(* Logix 5000 Program export ExtendedLaserCommands; software revision 21.03 *)

TYPE SETTIME :
STRUCT
   cmd : SETTIME_CMD;
   error : DINT;
END_STRUCT
END_TYPE

TYPE SETSYSTEMCOUNTER :
STRUCT
   cmd : SETSYSTEMCOUNTER_CMD;
   error : DINT;
END_STRUCT
END_TYPE

TYPE ExtendedLaserCommands :
STRUCT
   BUFFERCLEAR : NORES_CMD;
   BUFFERDATA : BUFFERDATA;
   BUFFERREVOKE : BUFFERREVOKE;
   GETBUFFERSTATUS : GETBUFFERSTATUS;
   GETCODINGFILE : GETCODINGFILE;
   SETCODINGFILE : SETCODINGFILE;
   GETCODINGLINE : GETINT;
   SETCODINGLINE : SETCODINGLINE;
   GETMSG24 : SIMPLECMD;
   GETMSG25 : MSG25;
   GETSYSTEMCOUNTER : GETSYSTEMCOUNTER;
   SETSYSTEMCOUNTER : SETSYSTEMCOUNTER;
   GETPRINTCOUNTER : GETINT;
   SETMAXCOUNTS : SETMAXCOUNTS;
   GETCO2ONPULSEOFFSET : GETINT;
   GETDATE : GETDATE;
   SETTIME : SETTIME;
   SETDATE : SETDATE;
   priv : LASER_PRIVATE_FIELDS;
END_STRUCT
END_TYPE

TYPE SIMPLECMD :
STRUCT
   cmd : EMPTY_CMD;
   res : LSTRING;
   error : DINT;
END_STRUCT
END_TYPE

TYPE GETDATE :
STRUCT
   cmd : EMPTY_CMD;
   res : GETDATE_RES;
   error : DINT;
END_STRUCT
END_TYPE

TYPE SETCODINGLINE :
STRUCT
   cmd : SETCODINGLINE_CMD;
   error : DINT;
END_STRUCT
END_TYPE

TYPE BUFFERDATA_CMD :
STRUCT
   ID : DINT;
   text1 : LSTRING;
   text2 : LSTRING;
   text3 : LSTRING;
   text4 : LSTRING;
   send : BOOL;
END_STRUCT
END_TYPE

TYPE LSTRING :   // string type
STRUCT
   LEN : DINT;
   DATA : SINT[400];
END_STRUCT
END_TYPE

TYPE SETDATE :
STRUCT
   cmd : SETDATE_CMD;
   error : DINT;
END_STRUCT
END_TYPE

TYPE BUFFERREVOKE :
STRUCT
   cmd : BUFFERREVOKE_CMD;
   error : DINT;
END_STRUCT
END_TYPE

TYPE LASER_PRIVATE_FIELDS :
STRUCT
   data : SINT[808];
   busy : BOOL;
END_STRUCT
END_TYPE

TYPE BUFFERREVOKE_CMD :
STRUCT
   function : LSTRING;
   parameter : DINT;
   send : BOOL;
END_STRUCT
END_TYPE

TYPE MSG25 :
STRUCT
   cmd : EMPTY_CMD;
   res : DINT;
   error : DINT;
END_STRUCT
END_TYPE

TYPE GETBUFFERSTATUS :
STRUCT
   cmd : EMPTY_CMD;
   res : DINT;
   error : DINT;
END_STRUCT
END_TYPE

TYPE GETINT_RES :
STRUCT
   value : DINT;
END_STRUCT
END_TYPE

TYPE SETCODINGFILE_CMD :
STRUCT
   filename : LSTRING;
   nCodes : LSTRING;
   send : BOOL;
END_STRUCT
END_TYPE

TYPE SETTIME_CMD :
STRUCT
   hour : DINT;
   minute : DINT;
   second : DINT;
   send : BOOL;
END_STRUCT
END_TYPE

TYPE EMPTY_CMD :
STRUCT
   send : BOOL;
END_STRUCT
END_TYPE

TYPE GETSYSTEMCOUNTER_CMD :
STRUCT
   id : DINT;
   send : BOOL;
END_STRUCT
END_TYPE

TYPE GETDATE_RES :
STRUCT
   hour : DINT;
   minute : DINT;
   second : DINT;
   year : DINT;
   month : DINT;
   day : DINT;
END_STRUCT
END_TYPE

TYPE GETCODINGFILE :
STRUCT
   cmd : EMPTY_CMD;
   res : GETCODINGFILE_RES;
   error : DINT;
END_STRUCT
END_TYPE

TYPE SETCODINGLINE_CMD :
STRUCT
   value : DINT;
   send : BOOL;
END_STRUCT
END_TYPE

TYPE BUFFERDATA :
STRUCT
   cmd : BUFFERDATA_CMD;
   error : DINT;
END_STRUCT
END_TYPE

TYPE GETSYSTEMCOUNTER_RES :
STRUCT
   id : DINT;
   value : DINT;
END_STRUCT
END_TYPE

TYPE SETSYSTEMCOUNTER_CMD :
STRUCT
   id : DINT;
   value : DINT;
   send : BOOL;
END_STRUCT
END_TYPE

TYPE SETMAXCOUNTS :
STRUCT
   cmd : SETMAXCOUNTS_CMD;
   error : DINT;
END_STRUCT
END_TYPE

TYPE GETINT :
STRUCT
   cmd : EMPTY_CMD;
   res : GETINT_RES;
   error : DINT;
END_STRUCT
END_TYPE

TYPE SETMAXCOUNTS_CMD :
STRUCT
   value : DINT;
   send : BOOL;
END_STRUCT
END_TYPE

TYPE SETDATE_CMD :
STRUCT
   hour : DINT;
   minute : DINT;
   second : DINT;
   year : DINT;
   month : DINT;
   day : DINT;
   send : BOOL;
END_STRUCT
END_TYPE

TYPE GETSYSTEMCOUNTER :
STRUCT
   cmd : GETSYSTEMCOUNTER_CMD;
   res : GETSYSTEMCOUNTER_RES;
   error : DINT;
END_STRUCT
END_TYPE

TYPE GETCODINGFILE_RES :
STRUCT
   filename : LSTRING;
   nCodes : DINT;
END_STRUCT
END_TYPE

TYPE SETCODINGFILE :
STRUCT
   cmd : SETCODINGFILE_CMD;
   error : DINT;
END_STRUCT
END_TYPE

TYPE NORES_CMD :
STRUCT
   cmd : EMPTY_CMD;
   error : DINT;
END_STRUCT
END_TYPE

ADD_ON_INSTRUCTION StrToArr   (* revision 1.0, vendor 1 *)
VAR_IN_OUT
   out : SINT[404]; {required}
   str : LSTRING; {required}
END_VAR
VAR_OUTPUT
   size : DINT; {access Read Only, required}
END_VAR

ROUTINE Logic   (* ladder *)
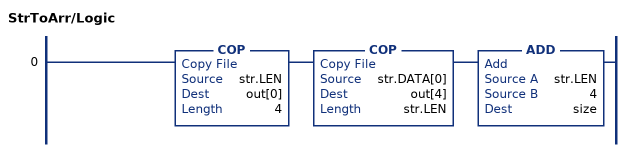
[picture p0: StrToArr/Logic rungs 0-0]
   0: COP(str.LEN,out[0],4)COP(str.DATA[0],out[4],str.LEN)ADD(str.LEN,4,size);
END_ROUTINE
END_ADD_ON_INSTRUCTION

ADD_ON_INSTRUCTION AppendStrs   (* revision 1.0, vendor 1 *)
VAR_IN_OUT
   str1 : LSTRING; {required}
   str2 : LSTRING; {required}
   out : SINT[808]; {required}
END_VAR
VAR_OUTPUT
   size : DINT; {access Read Only, required}
END_VAR
VAR
   cpy : StrToArr; {access None}
   n : DINT; {access None}
   offset : DINT; {access None}
   buf : SINT[404]; {access None}
END_VAR

ROUTINE Logic   (* ladder *)
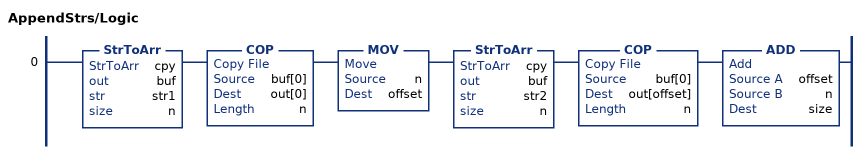
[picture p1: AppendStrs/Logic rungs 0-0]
   0: StrToArr(cpy,buf,str1,n)COP(buf[0],out[0],n)MOV(n,offset)StrToArr(cpy,buf,str2,n)COP(buf[0],out[offset],n)ADD(offset,n,size);
END_ROUTINE
END_ADD_ON_INSTRUCTION

ADD_ON_INSTRUCTION AppendStrs5   (* revision 1.0, vendor 1 *)
VAR_IN_OUT
   str1 : LSTRING; {required}
   str2 : LSTRING; {required}
   str3 : LSTRING; {required}
   str4 : LSTRING; {required}
   str5 : LSTRING; {required}
   out : SINT[808]; {required}
END_VAR
VAR_OUTPUT
   size : DINT; {access Read Only, required}
END_VAR
VAR_INPUT
   number_of_strings : DINT; {required}
   offset : DINT; {required}
END_VAR
VAR
   cpy : StrToArr; {access None}
   n : DINT; {access None}
   buf : SINT[404]; {access None}
END_VAR

ROUTINE Logic   (* ladder *)
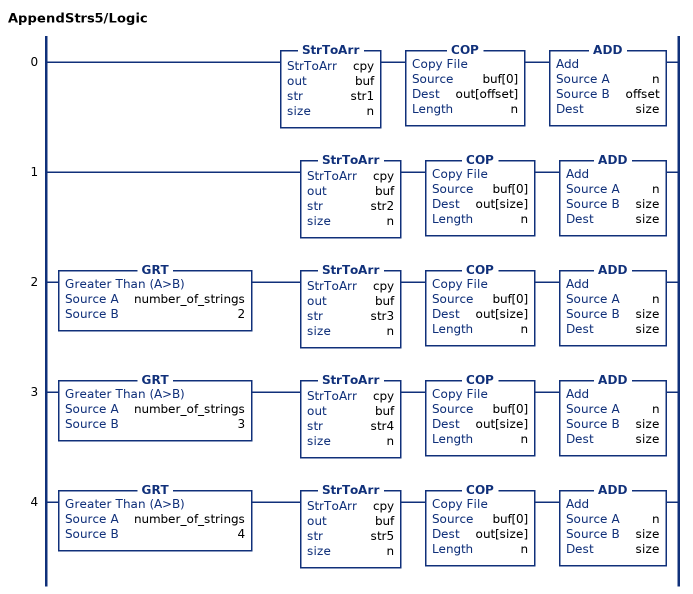
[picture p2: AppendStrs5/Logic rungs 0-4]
   0: StrToArr(cpy,buf,str1,n)COP(buf[0],out[offset],n)ADD(n,offset,size);
   1: StrToArr(cpy,buf,str2,n)COP(buf[0],out[size],n)ADD(n,size,size);
   2: GRT(number_of_strings,2)StrToArr(cpy,buf,str3,n)COP(buf[0],out[size],n)ADD(n,size,size);
   3: GRT(number_of_strings,3)StrToArr(cpy,buf,str4,n)COP(buf[0],out[size],n)ADD(n,size,size);
   4: GRT(number_of_strings,4)StrToArr(cpy,buf,str5,n)COP(buf[0],out[size],n)ADD(n,size,size);
END_ROUTINE
END_ADD_ON_INSTRUCTION

ADD_ON_INSTRUCTION ArrToStr   (* revision 1.0, vendor 1 *)
VAR_IN_OUT
   arr : SINT[404]; {required}
   out : LSTRING; {required}
END_VAR

ROUTINE Logic   (* ladder *)
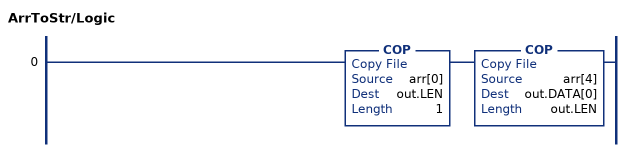
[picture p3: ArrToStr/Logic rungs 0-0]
   0: COP(arr[0],out.LEN,1)COP(arr[4],out.DATA[0],out.LEN);
END_ROUTINE
END_ADD_ON_INSTRUCTION

VAR_GLOBAL   (* controller tags *)
   Domino_internal_getprintcounter : MESSAGE;
        MessageParameters(MessageType := CIP Generic, ConnectedFlag := 2, ConnectionPath := DFSeries, ServiceCode := 16#0057, ObjectType := 16#0065, TargetObject := 1, LocalElement := DFSeriesExtended.priv, DestinationTag := DFSeriesExtended.priv)
   Domino_internal_setcodingline : MESSAGE;
        MessageParameters(MessageType := CIP Generic, RequestedLength := 4, ConnectedFlag := 2, ConnectionPath := DFSeries, ServiceCode := 16#0052, ObjectType := 16#0065, TargetObject := 1, LocalElement := DFSeriesExtended.priv, DestinationTag := DFSeriesExtended.priv)
   Domino_internal_setdate : MESSAGE;
        MessageParameters(MessageType := CIP Generic, RequestedLength := 24, ConnectedFlag := 2, ConnectionPath := DFSeries, ServiceCode := 16#005c, ObjectType := 16#0065, TargetObject := 1, LocalElement := DFSeriesExtended.priv, DestinationTag := DFSeriesExtended.priv)
   Domino_internal_getMSG25 : MESSAGE;
        MessageParameters(MessageType := CIP Generic, ConnectedFlag := 2, ConnectionPath := DFSeries, ServiceCode := 16#0054, ObjectType := 16#0065, TargetObject := 1, LocalElement := DFSeriesExtended.priv, DestinationTag := DFSeriesExtended.priv)
   Domino_internal_setcodingfile : MESSAGE;
        MessageParameters(MessageType := CIP Generic, RequestedLength := 1, ConnectedFlag := 2, ConnectionPath := DFSeries, ServiceCode := 16#0050, ObjectType := 16#0065, TargetObject := 1, LocalElement := DFSeriesExtended.priv, DestinationTag := DFSeriesExtended.priv)
   Domino_internal_setmaxcounts : MESSAGE;
        MessageParameters(MessageType := CIP Generic, RequestedLength := 4, ConnectedFlag := 2, ConnectionPath := DFSeries, ServiceCode := 16#0058, ObjectType := 16#0065, TargetObject := 1, LocalElement := DFSeriesExtended.priv, DestinationTag := DFSeriesExtended.priv)
   Domino_internal_getcodingfile : MESSAGE;
        MessageParameters(MessageType := CIP Generic, ConnectedFlag := 2, ConnectionPath := DFSeries, ServiceCode := 16#004f, ObjectType := 16#0065, TargetObject := 1, LocalElement := DFSeriesExtended.priv, DestinationTag := DFSeriesExtended.priv)
   Domino_internal_setsystemcounter : MESSAGE;
        MessageParameters(MessageType := CIP Generic, RequestedLength := 8, ConnectedFlag := 2, ConnectionPath := DFSeries, ServiceCode := 16#0056, ObjectType := 16#0065, TargetObject := 1, LocalElement := DFSeriesExtended.priv, DestinationTag := DFSeriesExtended.priv)
   Domino_internal_bufferclear : MESSAGE;
        MessageParameters(MessageType := CIP Generic, ConnectedFlag := 2, ConnectionPath := DFSeries, ServiceCode := 16#004b, ObjectType := 16#0065, TargetObject := 1, LocalElement := DFSeriesExtended.priv, DestinationTag := DFSeriesExtended.priv)
   DFSeriesExtended : ExtendedLaserCommands;
   Domino_internal_getcodingline : MESSAGE;
        MessageParameters(MessageType := CIP Generic, ConnectedFlag := 2, ConnectionPath := DFSeries, ServiceCode := 16#0051, ObjectType := 16#0065, TargetObject := 1, LocalElement := DFSeriesExtended.priv, DestinationTag := DFSeriesExtended.priv)
   Domino_internal_getco2onpulseoffset : MESSAGE;
        MessageParameters(MessageType := CIP Generic, ConnectedFlag := 2, ConnectionPath := DFSeries, ServiceCode := 16#0059, ObjectType := 16#0065, TargetObject := 1, LocalElement := DFSeriesExtended.priv, DestinationTag := DFSeriesExtended.priv)
   Domino_internal_getbufferstatus : MESSAGE;
        MessageParameters(MessageType := CIP Generic, ConnectedFlag := 2, ConnectionPath := DFSeries, ServiceCode := 16#004e, ObjectType := 16#0065, TargetObject := 1, LocalElement := DFSeriesExtended.priv, DestinationTag := DFSeriesExtended.priv)
   Domino_internal_bufferdata : MESSAGE;
        MessageParameters(MessageType := CIP Generic, RequestedLength := 1, ConnectedFlag := 2, ConnectionPath := DFSeries, ServiceCode := 16#004c, ObjectType := 16#0065, TargetObject := 1, LocalElement := DFSeriesExtended.priv, DestinationTag := DFSeriesExtended.priv)
   Domino_internal_getdate : MESSAGE;
        MessageParameters(MessageType := CIP Generic, ConnectedFlag := 2, ConnectionPath := DFSeries, ServiceCode := 16#005a, ObjectType := 16#0065, TargetObject := 1, LocalElement := DFSeriesExtended.priv, DestinationTag := DFSeriesExtended.priv)
   Domino_internal_settime : MESSAGE;
        MessageParameters(MessageType := CIP Generic, RequestedLength := 12, ConnectedFlag := 2, ConnectionPath := DFSeries, ServiceCode := 16#005b, ObjectType := 16#0065, TargetObject := 1, LocalElement := DFSeriesExtended.priv, DestinationTag := DFSeriesExtended.priv)
   Domino_internal_bufferrevoke : MESSAGE;
        MessageParameters(MessageType := CIP Generic, RequestedLength := 1, ConnectedFlag := 2, ConnectionPath := DFSeries, ServiceCode := 16#004d, ObjectType := 16#0065, TargetObject := 1, LocalElement := DFSeriesExtended.priv, DestinationTag := DFSeriesExtended.priv)
   Domino_internal_getsystemcounter : MESSAGE;
        MessageParameters(MessageType := CIP Generic, RequestedLength := 4, ConnectedFlag := 2, ConnectionPath := DFSeries, ServiceCode := 16#0055, ObjectType := 16#0065, TargetObject := 1, LocalElement := DFSeriesExtended.priv, DestinationTag := DFSeriesExtended.priv)
   Domino_internal_getMSG24 : MESSAGE;
        MessageParameters(MessageType := CIP Generic, ConnectedFlag := 2, ConnectionPath := DFSeries, ServiceCode := 16#0053, ObjectType := 16#0065, TargetObject := 1, LocalElement := DFSeriesExtended.priv, DestinationTag := DFSeriesExtended.priv)
END_VAR

PROGRAM ExtendedLaserCommands   (* main routine Main *)
VAR
   app : AppendStrs;
   app5 : AppendStrs5;
   toArr : StrToArr;
   toStr : ArrToStr;
END_VAR

ROUTINE Main   (* ladder *)
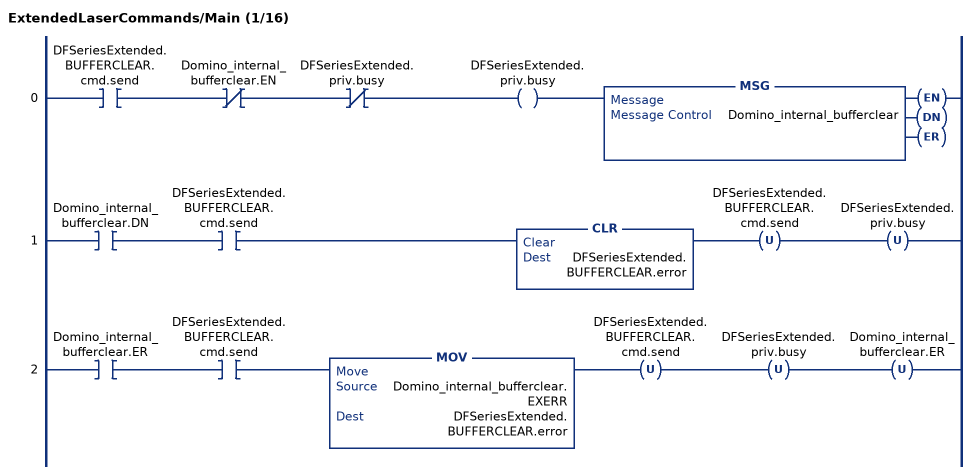
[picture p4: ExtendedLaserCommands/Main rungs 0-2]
   0: XIC(DFSeriesExtended.BUFFERCLEAR.cmd.send)XIO(Domino_internal_bufferclear.EN)XIO(DFSeriesExtended.priv.busy)OTE(DFSeriesExtended.priv.busy)MSG(Domino_internal_bufferclear);
   1: XIC(Domino_internal_bufferclear.DN)XIC(DFSeriesExtended.BUFFERCLEAR.cmd.send)CLR(DFSeriesExtended.BUFFERCLEAR.error)OTU(DFSeriesExtended.BUFFERCLEAR.cmd.send)OTU(DFSeriesExtended.priv.busy);
   2: XIC(Domino_internal_bufferclear.ER)XIC(DFSeriesExtended.BUFFERCLEAR.cmd.send)MOV(Domino_internal_bufferclear.EXERR,DFSeriesExtended.BUFFERCLEAR.error)OTU(DFSeriesExtended.BUFFERCLEAR.cmd.send)OTU(DFSeriesExtended.priv.busy)OTU(Domino_internal_bufferclear.ER);
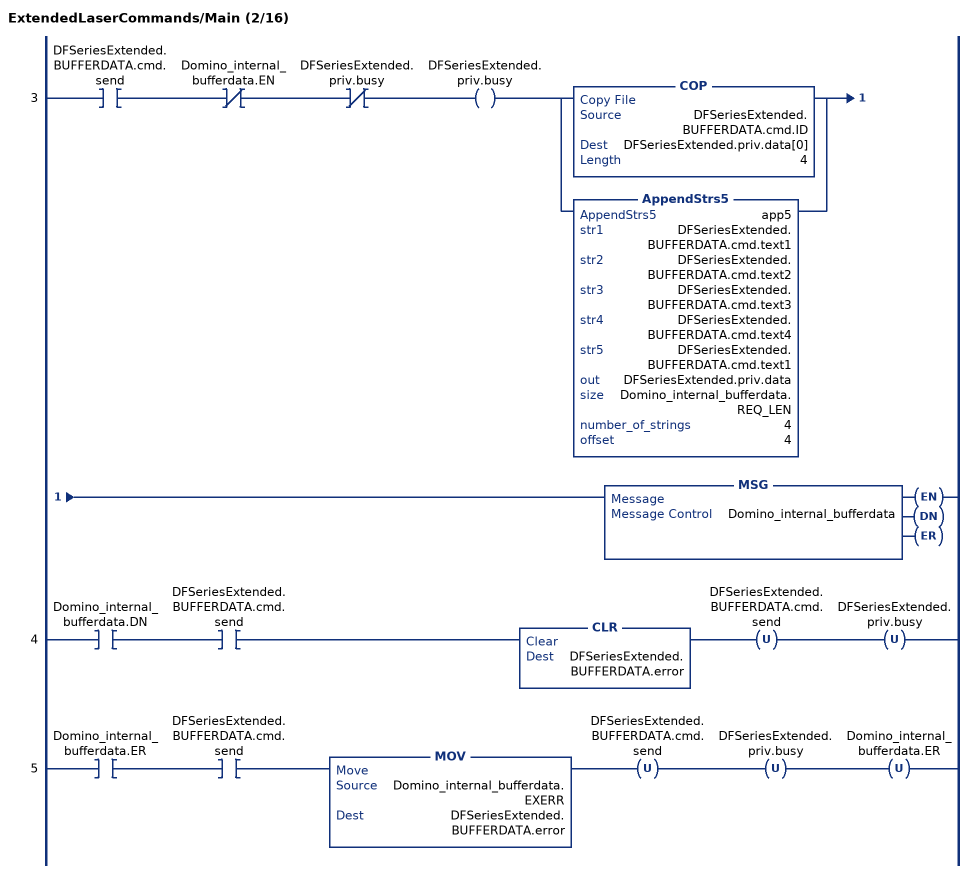
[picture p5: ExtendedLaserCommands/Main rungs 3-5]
   3: XIC(DFSeriesExtended.BUFFERDATA.cmd.send)XIO(Domino_internal_bufferdata.EN)XIO(DFSeriesExtended.priv.busy)OTE(DFSeriesExtended.priv.busy)[COP(DFSeriesExtended.BUFFERDATA.cmd.ID,DFSeriesExtended.priv.data[0],4) ,AppendStrs5(app5,DFSeriesExtended.BUFFERDATA.cmd.text1,DFSeriesExtended.BUFFERDATA.cmd.text2,DFSeriesExtended.BUFFERDATA.cmd.text3,DFSeriesExtended.BUFFERDATA.cmd.text4,DFSeriesExtended.BUFFERDATA.cmd.text1,DFSeriesExtended.priv.data,Domino_internal_bufferdata.REQ_LEN,4,4) ]MSG(Domino_internal_bufferdata);
   4: XIC(Domino_internal_bufferdata.DN)XIC(DFSeriesExtended.BUFFERDATA.cmd.send)CLR(DFSeriesExtended.BUFFERDATA.error)OTU(DFSeriesExtended.BUFFERDATA.cmd.send)OTU(DFSeriesExtended.priv.busy);
   5: XIC(Domino_internal_bufferdata.ER)XIC(DFSeriesExtended.BUFFERDATA.cmd.send)MOV(Domino_internal_bufferdata.EXERR,DFSeriesExtended.BUFFERDATA.error)OTU(DFSeriesExtended.BUFFERDATA.cmd.send)OTU(DFSeriesExtended.priv.busy)OTU(Domino_internal_bufferdata.ER);
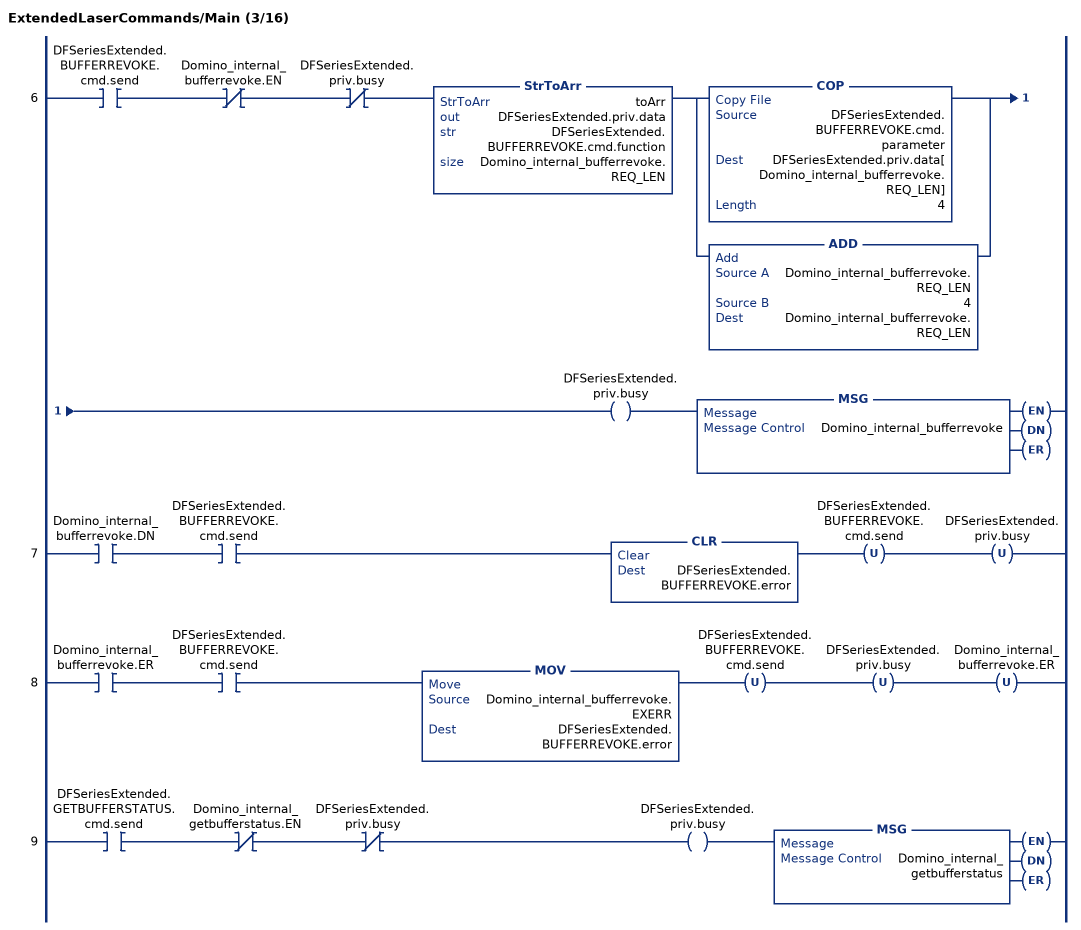
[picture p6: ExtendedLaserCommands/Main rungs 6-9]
   6: XIC(DFSeriesExtended.BUFFERREVOKE.cmd.send)XIO(Domino_internal_bufferrevoke.EN)XIO(DFSeriesExtended.priv.busy)StrToArr(toArr,DFSeriesExtended.priv.data,DFSeriesExtended.BUFFERREVOKE.cmd.function,Domino_internal_bufferrevoke.REQ_LEN)[COP(DFSeriesExtended.BUFFERREVOKE.cmd.parameter,DFSeriesExtended.priv.data[Domino_internal_bufferrevoke.REQ_LEN],4) ,ADD(Domino_internal_bufferrevoke.REQ_LEN,4,Domino_internal_bufferrevoke.REQ_LEN) ]OTE(DFSeriesExtended.priv.busy)MSG(Domino_internal_bufferrevoke);
   7: XIC(Domino_internal_bufferrevoke.DN)XIC(DFSeriesExtended.BUFFERREVOKE.cmd.send)CLR(DFSeriesExtended.BUFFERREVOKE.error)OTU(DFSeriesExtended.BUFFERREVOKE.cmd.send)OTU(DFSeriesExtended.priv.busy);
   8: XIC(Domino_internal_bufferrevoke.ER)XIC(DFSeriesExtended.BUFFERREVOKE.cmd.send)MOV(Domino_internal_bufferrevoke.EXERR,DFSeriesExtended.BUFFERREVOKE.error)OTU(DFSeriesExtended.BUFFERREVOKE.cmd.send)OTU(DFSeriesExtended.priv.busy)OTU(Domino_internal_bufferrevoke.ER);
   9: XIC(DFSeriesExtended.GETBUFFERSTATUS.cmd.send)XIO(Domino_internal_getbufferstatus.EN)XIO(DFSeriesExtended.priv.busy)OTE(DFSeriesExtended.priv.busy)MSG(Domino_internal_getbufferstatus);
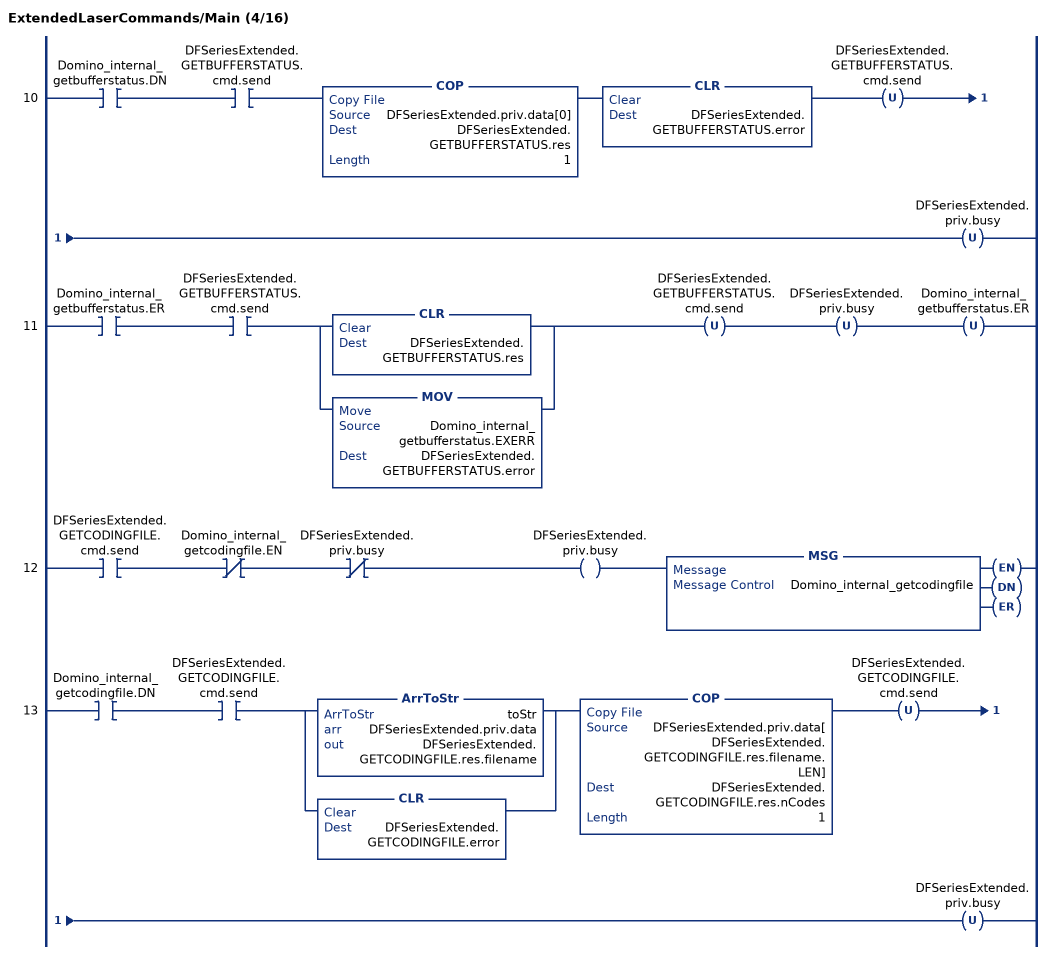
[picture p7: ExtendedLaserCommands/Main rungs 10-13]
   10: XIC(Domino_internal_getbufferstatus.DN)XIC(DFSeriesExtended.GETBUFFERSTATUS.cmd.send)COP(DFSeriesExtended.priv.data[0],DFSeriesExtended.GETBUFFERSTATUS.res,1)CLR(DFSeriesExtended.GETBUFFERSTATUS.error)OTU(DFSeriesExtended.GETBUFFERSTATUS.cmd.send)OTU(DFSeriesExtended.priv.busy);
   11: XIC(Domino_internal_getbufferstatus.ER)XIC(DFSeriesExtended.GETBUFFERSTATUS.cmd.send)[CLR(DFSeriesExtended.GETBUFFERSTATUS.res) ,MOV(Domino_internal_getbufferstatus.EXERR,DFSeriesExtended.GETBUFFERSTATUS.error) ]OTU(DFSeriesExtended.GETBUFFERSTATUS.cmd.send)OTU(DFSeriesExtended.priv.busy)OTU(Domino_internal_getbufferstatus.ER);
   12: XIC(DFSeriesExtended.GETCODINGFILE.cmd.send)XIO(Domino_internal_getcodingfile.EN)XIO(DFSeriesExtended.priv.busy)OTE(DFSeriesExtended.priv.busy)MSG(Domino_internal_getcodingfile);
   13: XIC(Domino_internal_getcodingfile.DN)XIC(DFSeriesExtended.GETCODINGFILE.cmd.send)[ArrToStr(toStr,DFSeriesExtended.priv.data,DFSeriesExtended.GETCODINGFILE.res.filename) ,CLR(DFSeriesExtended.GETCODINGFILE.error) ]COP(DFSeriesExtended.priv.data[DFSeriesExtended.GETCODINGFILE.res.filename.LEN],DFSeriesExtended.GETCODINGFILE.res.nCodes,1)OTU(DFSeriesExtended.GETCODINGFILE.cmd.send)OTU(DFSeriesExtended.priv.busy);
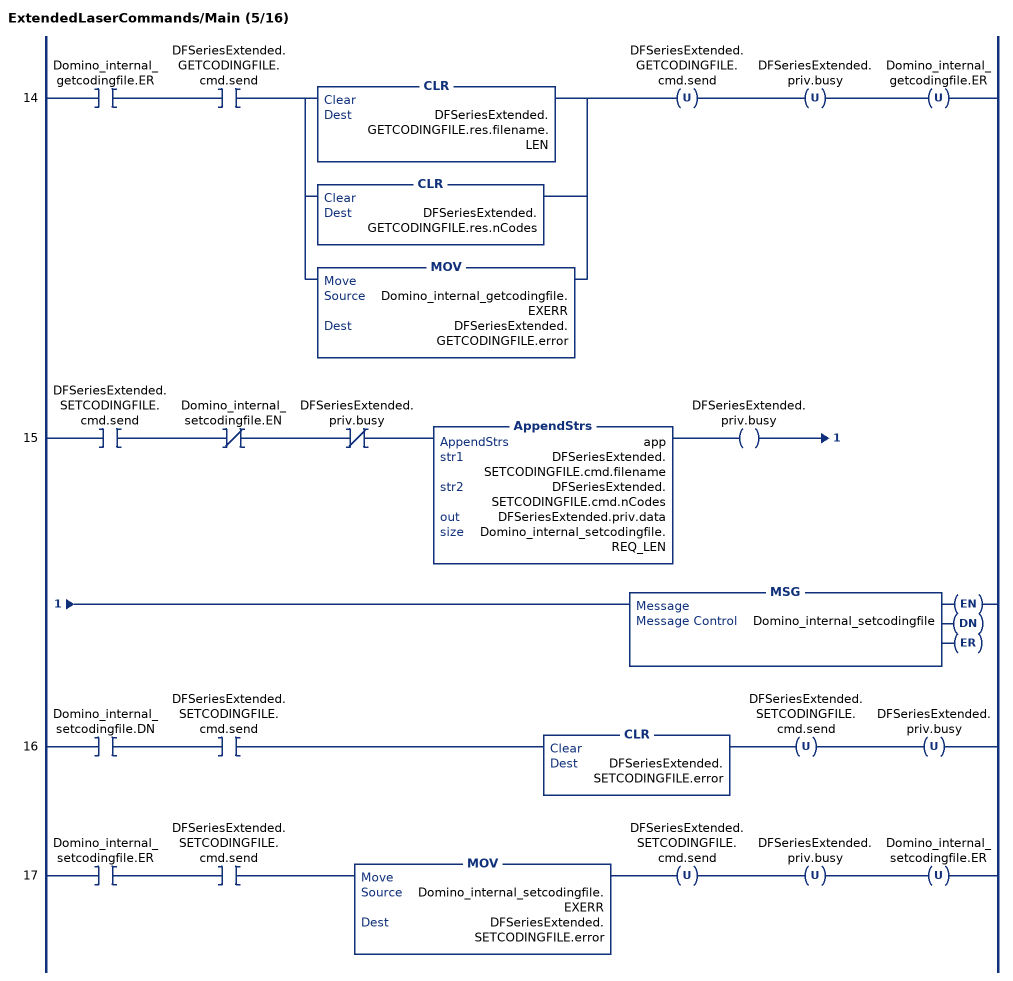
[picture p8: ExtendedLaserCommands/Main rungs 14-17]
   14: XIC(Domino_internal_getcodingfile.ER)XIC(DFSeriesExtended.GETCODINGFILE.cmd.send)[CLR(DFSeriesExtended.GETCODINGFILE.res.filename.LEN) ,CLR(DFSeriesExtended.GETCODINGFILE.res.nCodes) ,MOV(Domino_internal_getcodingfile.EXERR,DFSeriesExtended.GETCODINGFILE.error) ]OTU(DFSeriesExtended.GETCODINGFILE.cmd.send)OTU(DFSeriesExtended.priv.busy)OTU(Domino_internal_getcodingfile.ER);
   15: XIC(DFSeriesExtended.SETCODINGFILE.cmd.send)XIO(Domino_internal_setcodingfile.EN)XIO(DFSeriesExtended.priv.busy)AppendStrs(app,DFSeriesExtended.SETCODINGFILE.cmd.filename,DFSeriesExtended.SETCODINGFILE.cmd.nCodes,DFSeriesExtended.priv.data,Domino_internal_setcodingfile.REQ_LEN)OTE(DFSeriesExtended.priv.busy)MSG(Domino_internal_setcodingfile);
   16: XIC(Domino_internal_setcodingfile.DN)XIC(DFSeriesExtended.SETCODINGFILE.cmd.send)CLR(DFSeriesExtended.SETCODINGFILE.error)OTU(DFSeriesExtended.SETCODINGFILE.cmd.send)OTU(DFSeriesExtended.priv.busy);
   17: XIC(Domino_internal_setcodingfile.ER)XIC(DFSeriesExtended.SETCODINGFILE.cmd.send)MOV(Domino_internal_setcodingfile.EXERR,DFSeriesExtended.SETCODINGFILE.error)OTU(DFSeriesExtended.SETCODINGFILE.cmd.send)OTU(DFSeriesExtended.priv.busy)OTU(Domino_internal_setcodingfile.ER);
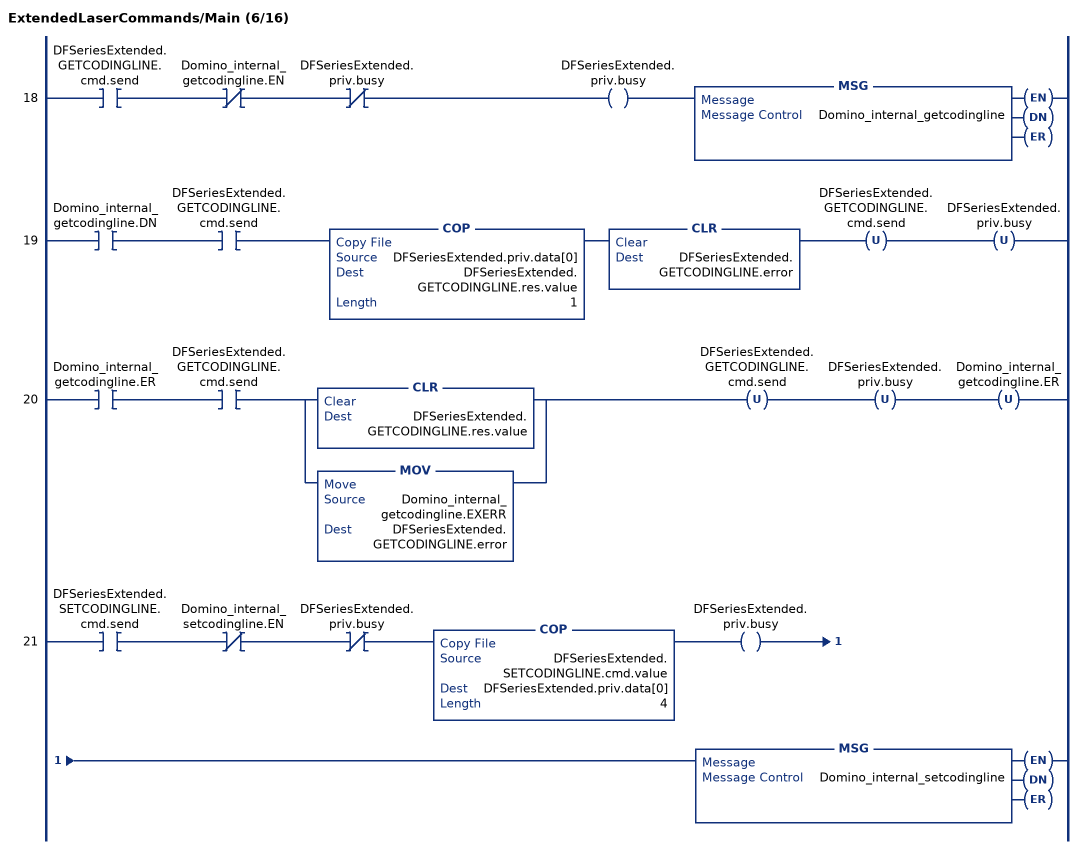
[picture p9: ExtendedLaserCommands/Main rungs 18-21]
   18: XIC(DFSeriesExtended.GETCODINGLINE.cmd.send)XIO(Domino_internal_getcodingline.EN)XIO(DFSeriesExtended.priv.busy)OTE(DFSeriesExtended.priv.busy)MSG(Domino_internal_getcodingline);
   19: XIC(Domino_internal_getcodingline.DN)XIC(DFSeriesExtended.GETCODINGLINE.cmd.send)COP(DFSeriesExtended.priv.data[0],DFSeriesExtended.GETCODINGLINE.res.value,1)CLR(DFSeriesExtended.GETCODINGLINE.error)OTU(DFSeriesExtended.GETCODINGLINE.cmd.send)OTU(DFSeriesExtended.priv.busy);
   20: XIC(Domino_internal_getcodingline.ER)XIC(DFSeriesExtended.GETCODINGLINE.cmd.send)[CLR(DFSeriesExtended.GETCODINGLINE.res.value) ,MOV(Domino_internal_getcodingline.EXERR,DFSeriesExtended.GETCODINGLINE.error) ]OTU(DFSeriesExtended.GETCODINGLINE.cmd.send)OTU(DFSeriesExtended.priv.busy)OTU(Domino_internal_getcodingline.ER);
   21: XIC(DFSeriesExtended.SETCODINGLINE.cmd.send)XIO(Domino_internal_setcodingline.EN)XIO(DFSeriesExtended.priv.busy)COP(DFSeriesExtended.SETCODINGLINE.cmd.value,DFSeriesExtended.priv.data[0],4)OTE(DFSeriesExtended.priv.busy)MSG(Domino_internal_setcodingline);
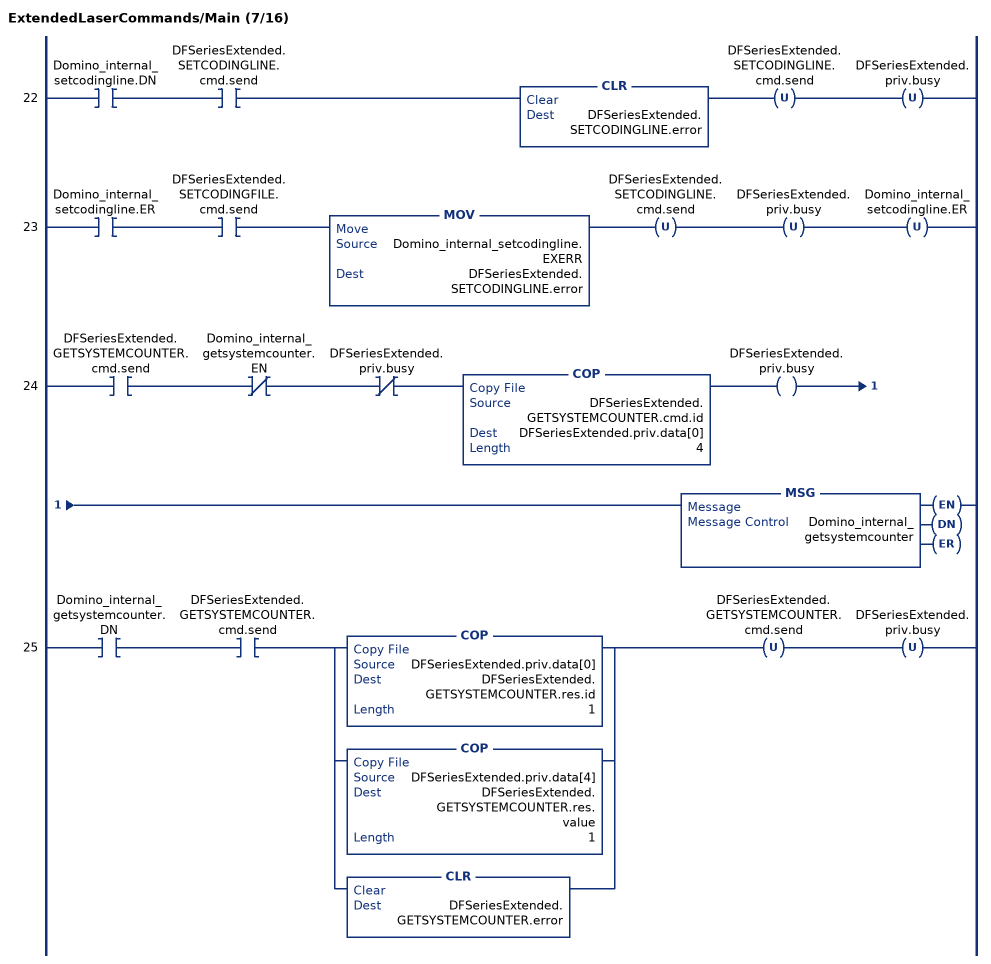
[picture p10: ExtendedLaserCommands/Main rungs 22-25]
   22: XIC(Domino_internal_setcodingline.DN)XIC(DFSeriesExtended.SETCODINGLINE.cmd.send)CLR(DFSeriesExtended.SETCODINGLINE.error)OTU(DFSeriesExtended.SETCODINGLINE.cmd.send)OTU(DFSeriesExtended.priv.busy);
   23: XIC(Domino_internal_setcodingline.ER)XIC(DFSeriesExtended.SETCODINGFILE.cmd.send)MOV(Domino_internal_setcodingline.EXERR,DFSeriesExtended.SETCODINGLINE.error)OTU(DFSeriesExtended.SETCODINGLINE.cmd.send)OTU(DFSeriesExtended.priv.busy)OTU(Domino_internal_setcodingline.ER);
   24: XIC(DFSeriesExtended.GETSYSTEMCOUNTER.cmd.send)XIO(Domino_internal_getsystemcounter.EN)XIO(DFSeriesExtended.priv.busy)COP(DFSeriesExtended.GETSYSTEMCOUNTER.cmd.id,DFSeriesExtended.priv.data[0],4)OTE(DFSeriesExtended.priv.busy)MSG(Domino_internal_getsystemcounter);
   25: XIC(Domino_internal_getsystemcounter.DN)XIC(DFSeriesExtended.GETSYSTEMCOUNTER.cmd.send)[COP(DFSeriesExtended.priv.data[0],DFSeriesExtended.GETSYSTEMCOUNTER.res.id,1) ,COP(DFSeriesExtended.priv.data[4],DFSeriesExtended.GETSYSTEMCOUNTER.res.value,1) ,CLR(DFSeriesExtended.GETSYSTEMCOUNTER.error) ]OTU(DFSeriesExtended.GETSYSTEMCOUNTER.cmd.send)OTU(DFSeriesExtended.priv.busy);
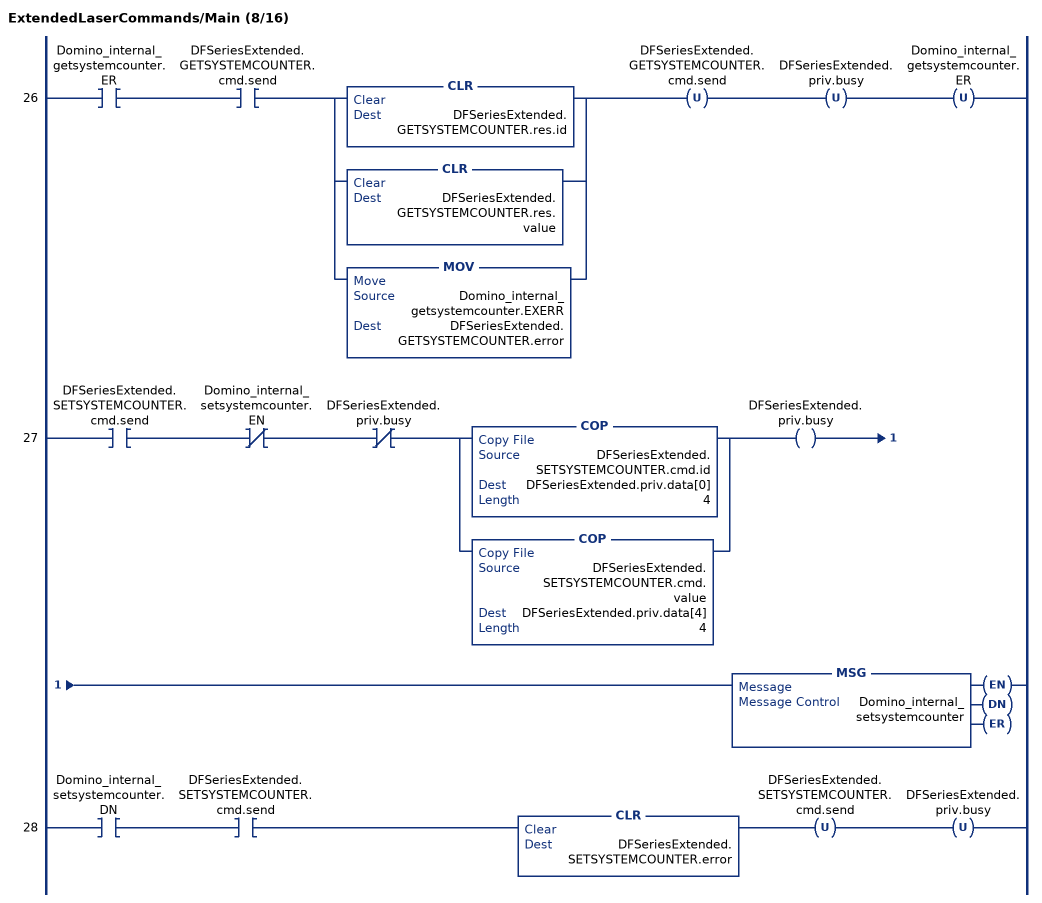
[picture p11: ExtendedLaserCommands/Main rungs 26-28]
   26: XIC(Domino_internal_getsystemcounter.ER)XIC(DFSeriesExtended.GETSYSTEMCOUNTER.cmd.send)[CLR(DFSeriesExtended.GETSYSTEMCOUNTER.res.id) ,CLR(DFSeriesExtended.GETSYSTEMCOUNTER.res.value) ,MOV(Domino_internal_getsystemcounter.EXERR,DFSeriesExtended.GETSYSTEMCOUNTER.error) ]OTU(DFSeriesExtended.GETSYSTEMCOUNTER.cmd.send)OTU(DFSeriesExtended.priv.busy)OTU(Domino_internal_getsystemcounter.ER);
   27: XIC(DFSeriesExtended.SETSYSTEMCOUNTER.cmd.send)XIO(Domino_internal_setsystemcounter.EN)XIO(DFSeriesExtended.priv.busy)[COP(DFSeriesExtended.SETSYSTEMCOUNTER.cmd.id,DFSeriesExtended.priv.data[0],4) ,COP(DFSeriesExtended.SETSYSTEMCOUNTER.cmd.value,DFSeriesExtended.priv.data[4],4) ]OTE(DFSeriesExtended.priv.busy)MSG(Domino_internal_setsystemcounter);
   28: XIC(Domino_internal_setsystemcounter.DN)XIC(DFSeriesExtended.SETSYSTEMCOUNTER.cmd.send)CLR(DFSeriesExtended.SETSYSTEMCOUNTER.error)OTU(DFSeriesExtended.SETSYSTEMCOUNTER.cmd.send)OTU(DFSeriesExtended.priv.busy);
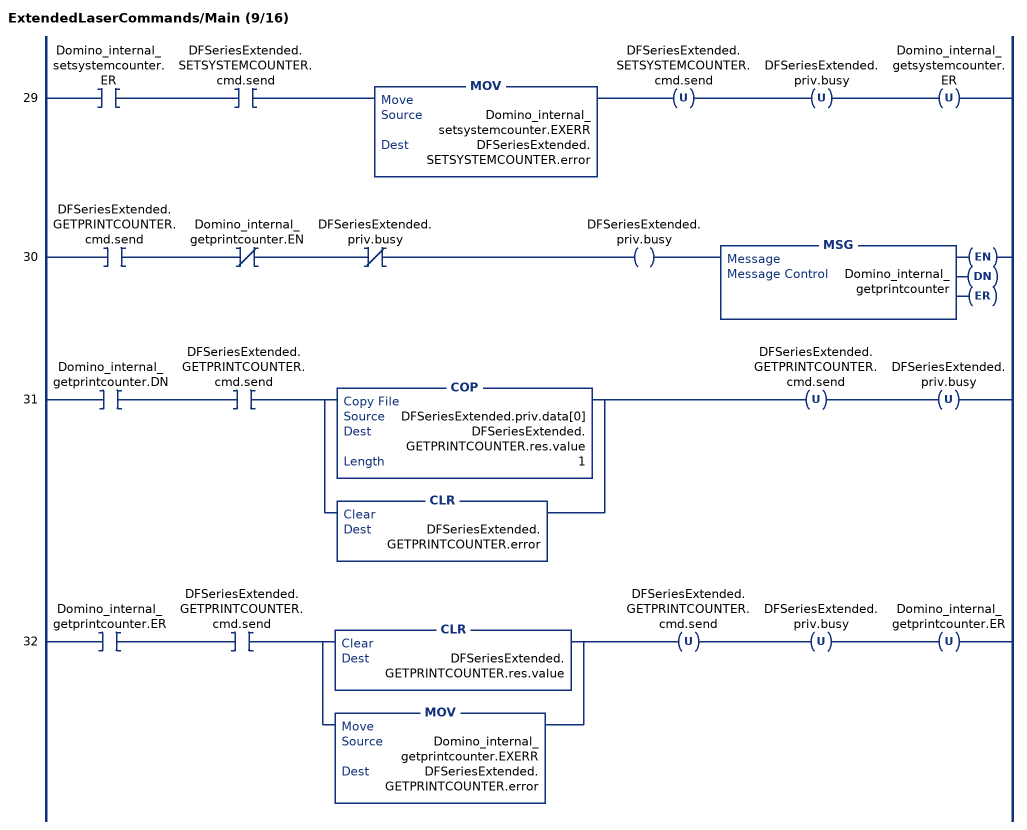
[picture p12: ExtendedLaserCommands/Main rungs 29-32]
   29: XIC(Domino_internal_setsystemcounter.ER)XIC(DFSeriesExtended.SETSYSTEMCOUNTER.cmd.send)MOV(Domino_internal_setsystemcounter.EXERR,DFSeriesExtended.SETSYSTEMCOUNTER.error)OTU(DFSeriesExtended.SETSYSTEMCOUNTER.cmd.send)OTU(DFSeriesExtended.priv.busy)OTU(Domino_internal_getsystemcounter.ER);
   30: XIC(DFSeriesExtended.GETPRINTCOUNTER.cmd.send)XIO(Domino_internal_getprintcounter.EN)XIO(DFSeriesExtended.priv.busy)OTE(DFSeriesExtended.priv.busy)MSG(Domino_internal_getprintcounter);
   31: XIC(Domino_internal_getprintcounter.DN)XIC(DFSeriesExtended.GETPRINTCOUNTER.cmd.send)[COP(DFSeriesExtended.priv.data[0],DFSeriesExtended.GETPRINTCOUNTER.res.value,1) ,CLR(DFSeriesExtended.GETPRINTCOUNTER.error) ]OTU(DFSeriesExtended.GETPRINTCOUNTER.cmd.send)OTU(DFSeriesExtended.priv.busy);
   32: XIC(Domino_internal_getprintcounter.ER)XIC(DFSeriesExtended.GETPRINTCOUNTER.cmd.send)[CLR(DFSeriesExtended.GETPRINTCOUNTER.res.value) ,MOV(Domino_internal_getprintcounter.EXERR,DFSeriesExtended.GETPRINTCOUNTER.error) ]OTU(DFSeriesExtended.GETPRINTCOUNTER.cmd.send)OTU(DFSeriesExtended.priv.busy)OTU(Domino_internal_getprintcounter.ER);
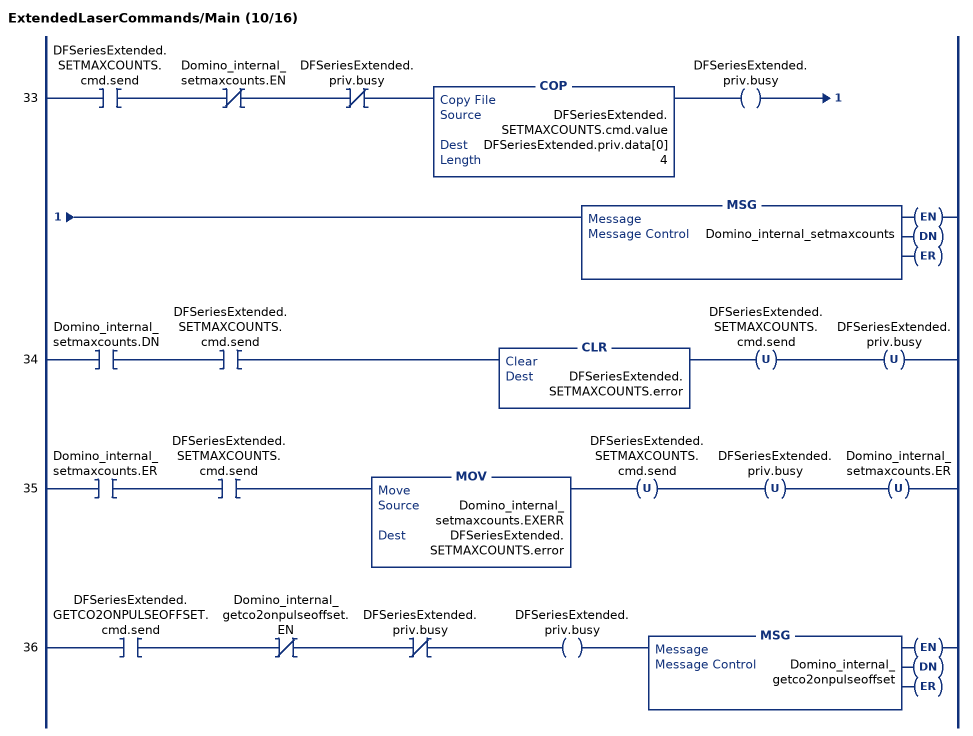
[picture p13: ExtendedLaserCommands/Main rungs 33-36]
   33: XIC(DFSeriesExtended.SETMAXCOUNTS.cmd.send)XIO(Domino_internal_setmaxcounts.EN)XIO(DFSeriesExtended.priv.busy)COP(DFSeriesExtended.SETMAXCOUNTS.cmd.value,DFSeriesExtended.priv.data[0],4)OTE(DFSeriesExtended.priv.busy)MSG(Domino_internal_setmaxcounts);
   34: XIC(Domino_internal_setmaxcounts.DN)XIC(DFSeriesExtended.SETMAXCOUNTS.cmd.send)CLR(DFSeriesExtended.SETMAXCOUNTS.error)OTU(DFSeriesExtended.SETMAXCOUNTS.cmd.send)OTU(DFSeriesExtended.priv.busy);
   35: XIC(Domino_internal_setmaxcounts.ER)XIC(DFSeriesExtended.SETMAXCOUNTS.cmd.send)MOV(Domino_internal_setmaxcounts.EXERR,DFSeriesExtended.SETMAXCOUNTS.error)OTU(DFSeriesExtended.SETMAXCOUNTS.cmd.send)OTU(DFSeriesExtended.priv.busy)OTU(Domino_internal_setmaxcounts.ER);
   36: XIC(DFSeriesExtended.GETCO2ONPULSEOFFSET.cmd.send)XIO(Domino_internal_getco2onpulseoffset.EN)XIO(DFSeriesExtended.priv.busy)OTE(DFSeriesExtended.priv.busy)MSG(Domino_internal_getco2onpulseoffset);
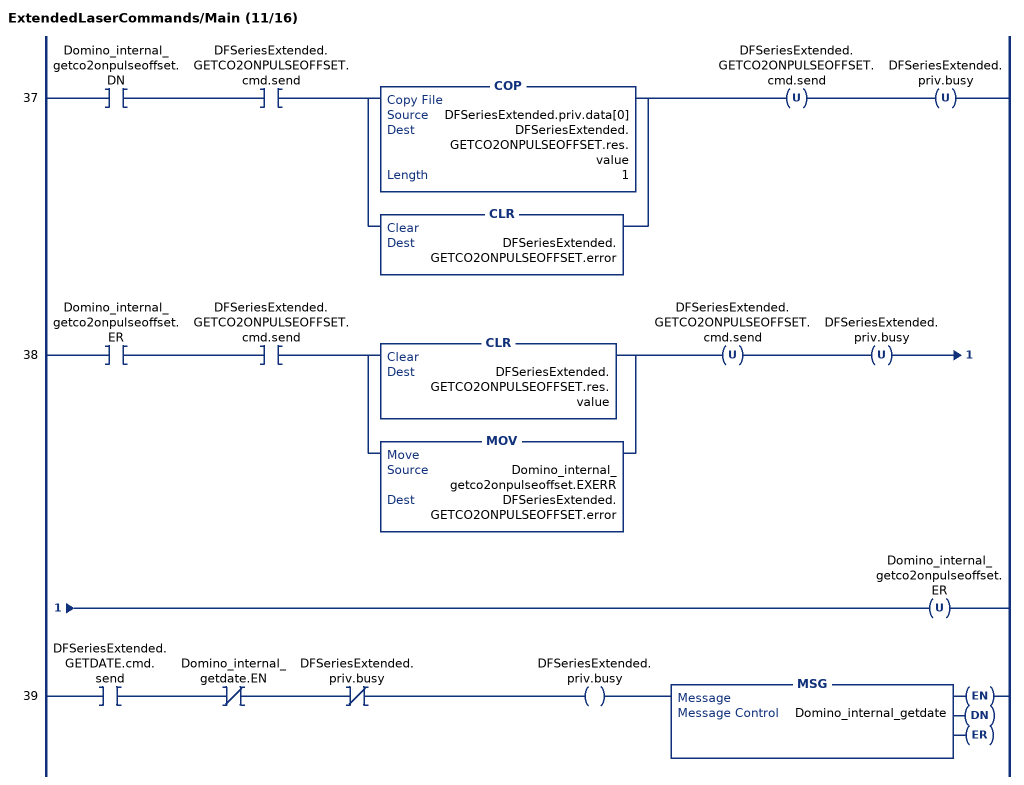
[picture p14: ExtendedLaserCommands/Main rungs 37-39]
   37: XIC(Domino_internal_getco2onpulseoffset.DN)XIC(DFSeriesExtended.GETCO2ONPULSEOFFSET.cmd.send)[COP(DFSeriesExtended.priv.data[0],DFSeriesExtended.GETCO2ONPULSEOFFSET.res.value,1) ,CLR(DFSeriesExtended.GETCO2ONPULSEOFFSET.error) ]OTU(DFSeriesExtended.GETCO2ONPULSEOFFSET.cmd.send)OTU(DFSeriesExtended.priv.busy);
   38: XIC(Domino_internal_getco2onpulseoffset.ER)XIC(DFSeriesExtended.GETCO2ONPULSEOFFSET.cmd.send)[CLR(DFSeriesExtended.GETCO2ONPULSEOFFSET.res.value) ,MOV(Domino_internal_getco2onpulseoffset.EXERR,DFSeriesExtended.GETCO2ONPULSEOFFSET.error) ]OTU(DFSeriesExtended.GETCO2ONPULSEOFFSET.cmd.send)OTU(DFSeriesExtended.priv.busy)OTU(Domino_internal_getco2onpulseoffset.ER);
   39: XIC(DFSeriesExtended.GETDATE.cmd.send)XIO(Domino_internal_getdate.EN)XIO(DFSeriesExtended.priv.busy)OTE(DFSeriesExtended.priv.busy)MSG(Domino_internal_getdate);
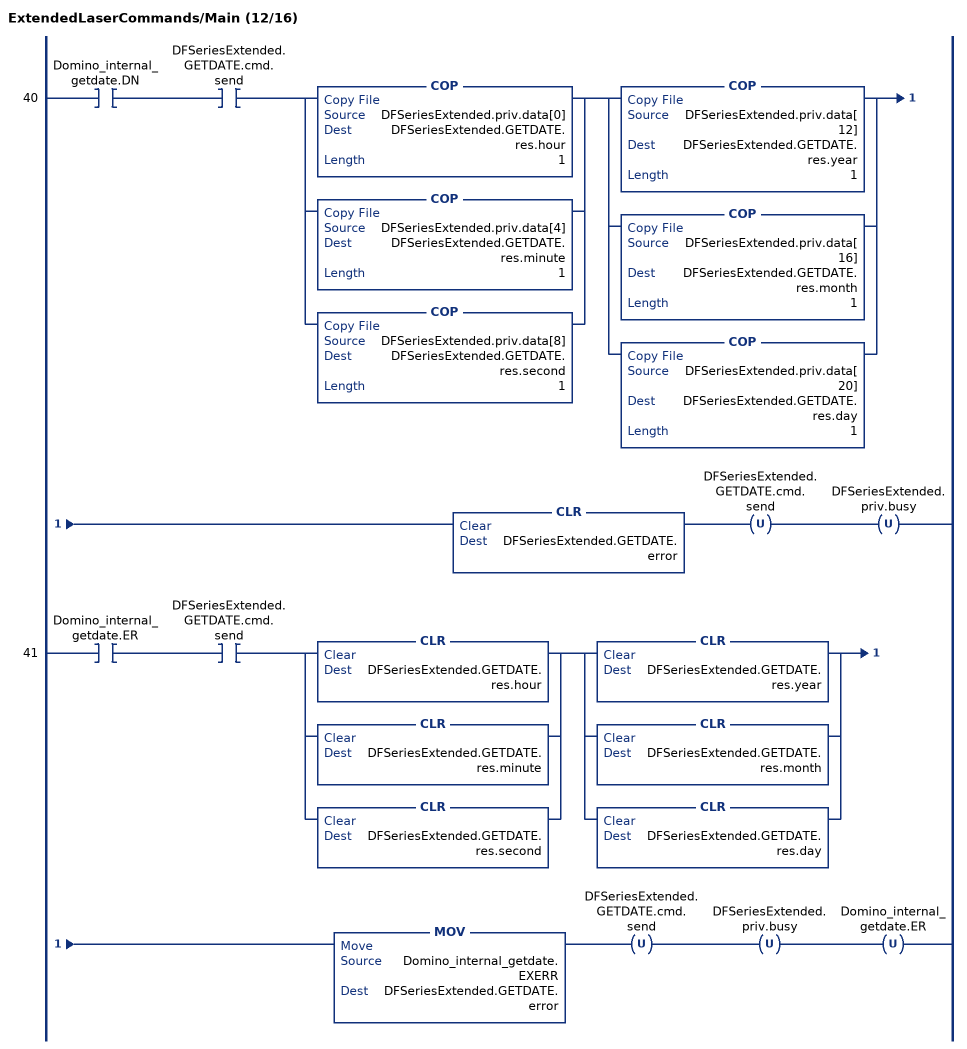
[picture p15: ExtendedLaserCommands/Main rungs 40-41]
   40: XIC(Domino_internal_getdate.DN)XIC(DFSeriesExtended.GETDATE.cmd.send)[COP(DFSeriesExtended.priv.data[0],DFSeriesExtended.GETDATE.res.hour,1) ,COP(DFSeriesExtended.priv.data[4],DFSeriesExtended.GETDATE.res.minute,1) ,COP(DFSeriesExtended.priv.data[8],DFSeriesExtended.GETDATE.res.second,1) ][COP(DFSeriesExtended.priv.data[12],DFSeriesExtended.GETDATE.res.year,1) ,COP(DFSeriesExtended.priv.data[16],DFSeriesExtended.GETDATE.res.month,1) ,COP(DFSeriesExtended.priv.data[20],DFSeriesExtended.GETDATE.res.day,1) ]CLR(DFSeriesExtended.GETDATE.error)OTU(DFSeriesExtended.GETDATE.cmd.send)OTU(DFSeriesExtended.priv.busy);
   41: XIC(Domino_internal_getdate.ER)XIC(DFSeriesExtended.GETDATE.cmd.send)[CLR(DFSeriesExtended.GETDATE.res.hour) ,CLR(DFSeriesExtended.GETDATE.res.minute) ,CLR(DFSeriesExtended.GETDATE.res.second) ][CLR(DFSeriesExtended.GETDATE.res.year) ,CLR(DFSeriesExtended.GETDATE.res.month) ,CLR(DFSeriesExtended.GETDATE.res.day) ]MOV(Domino_internal_getdate.EXERR,DFSeriesExtended.GETDATE.error)OTU(DFSeriesExtended.GETDATE.cmd.send)OTU(DFSeriesExtended.priv.busy)OTU(Domino_internal_getdate.ER);
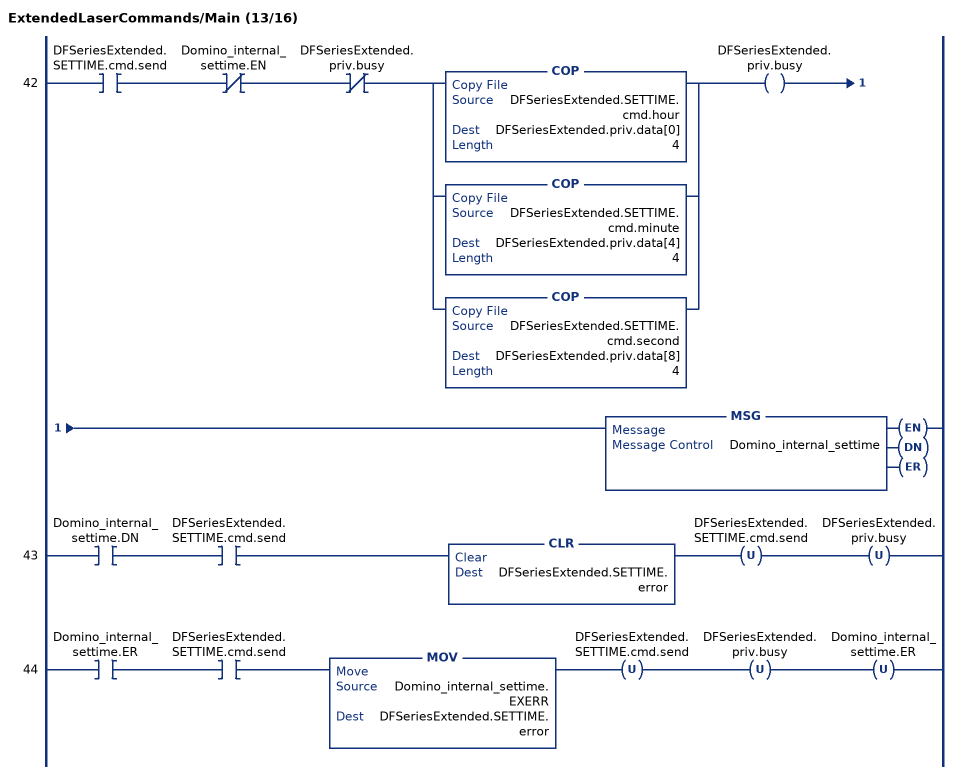
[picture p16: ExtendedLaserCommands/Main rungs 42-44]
   42: XIC(DFSeriesExtended.SETTIME.cmd.send)XIO(Domino_internal_settime.EN)XIO(DFSeriesExtended.priv.busy)[COP(DFSeriesExtended.SETTIME.cmd.hour,DFSeriesExtended.priv.data[0],4) ,COP(DFSeriesExtended.SETTIME.cmd.minute,DFSeriesExtended.priv.data[4],4) ,COP(DFSeriesExtended.SETTIME.cmd.second,DFSeriesExtended.priv.data[8],4) ]OTE(DFSeriesExtended.priv.busy)MSG(Domino_internal_settime);
   43: XIC(Domino_internal_settime.DN)XIC(DFSeriesExtended.SETTIME.cmd.send)CLR(DFSeriesExtended.SETTIME.error)OTU(DFSeriesExtended.SETTIME.cmd.send)OTU(DFSeriesExtended.priv.busy);
   44: XIC(Domino_internal_settime.ER)XIC(DFSeriesExtended.SETTIME.cmd.send)MOV(Domino_internal_settime.EXERR,DFSeriesExtended.SETTIME.error)OTU(DFSeriesExtended.SETTIME.cmd.send)OTU(DFSeriesExtended.priv.busy)OTU(Domino_internal_settime.ER);
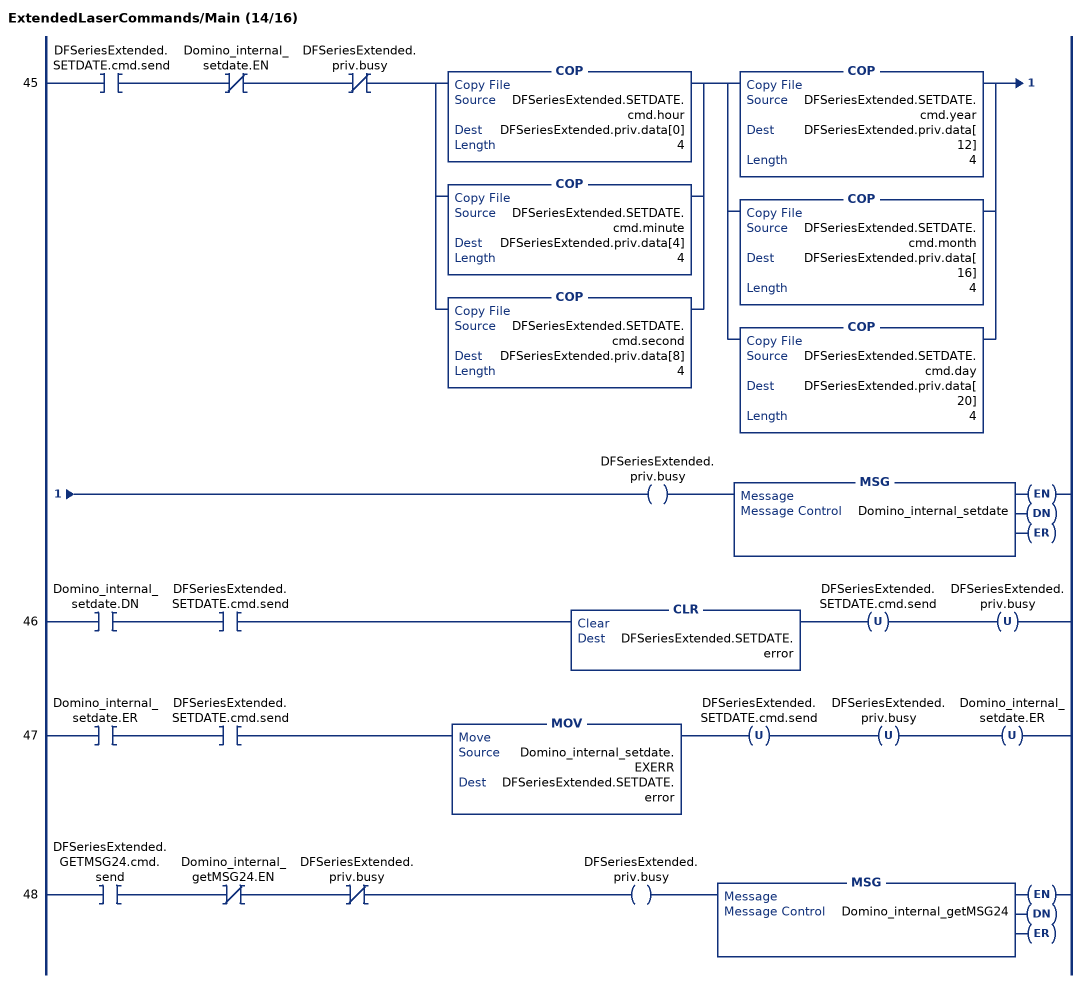
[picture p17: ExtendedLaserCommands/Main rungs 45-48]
   45: XIC(DFSeriesExtended.SETDATE.cmd.send)XIO(Domino_internal_setdate.EN)XIO(DFSeriesExtended.priv.busy)[COP(DFSeriesExtended.SETDATE.cmd.hour,DFSeriesExtended.priv.data[0],4) ,COP(DFSeriesExtended.SETDATE.cmd.minute,DFSeriesExtended.priv.data[4],4) ,COP(DFSeriesExtended.SETDATE.cmd.second,DFSeriesExtended.priv.data[8],4) ][COP(DFSeriesExtended.SETDATE.cmd.year,DFSeriesExtended.priv.data[12],4) ,COP(DFSeriesExtended.SETDATE.cmd.month,DFSeriesExtended.priv.data[16],4) ,COP(DFSeriesExtended.SETDATE.cmd.day,DFSeriesExtended.priv.data[20],4) ]OTE(DFSeriesExtended.priv.busy)MSG(Domino_internal_setdate);
   46: XIC(Domino_internal_setdate.DN)XIC(DFSeriesExtended.SETDATE.cmd.send)CLR(DFSeriesExtended.SETDATE.error)OTU(DFSeriesExtended.SETDATE.cmd.send)OTU(DFSeriesExtended.priv.busy);
   47: XIC(Domino_internal_setdate.ER)XIC(DFSeriesExtended.SETDATE.cmd.send)MOV(Domino_internal_setdate.EXERR,DFSeriesExtended.SETDATE.error)OTU(DFSeriesExtended.SETDATE.cmd.send)OTU(DFSeriesExtended.priv.busy)OTU(Domino_internal_setdate.ER);
   48: XIC(DFSeriesExtended.GETMSG24.cmd.send)XIO(Domino_internal_getMSG24.EN)XIO(DFSeriesExtended.priv.busy)OTE(DFSeriesExtended.priv.busy)MSG(Domino_internal_getMSG24);
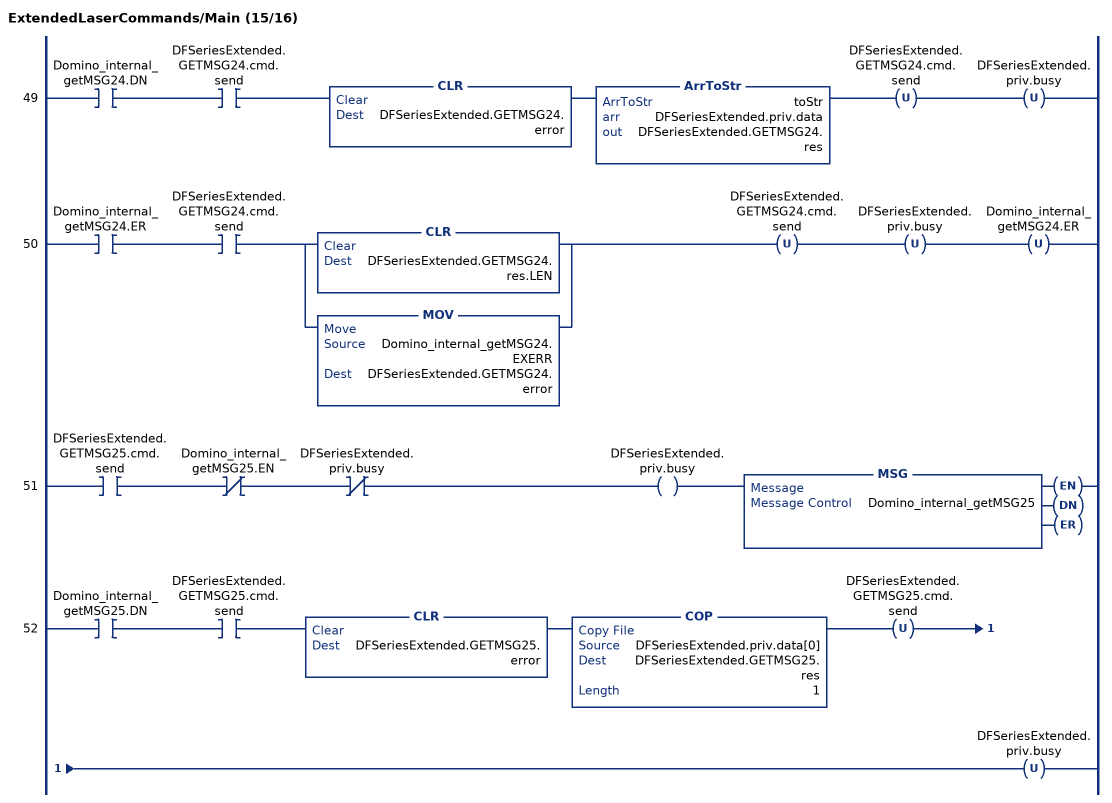
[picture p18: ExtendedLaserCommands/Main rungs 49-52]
   49: XIC(Domino_internal_getMSG24.DN)XIC(DFSeriesExtended.GETMSG24.cmd.send)CLR(DFSeriesExtended.GETMSG24.error)ArrToStr(toStr,DFSeriesExtended.priv.data,DFSeriesExtended.GETMSG24.res)OTU(DFSeriesExtended.GETMSG24.cmd.send)OTU(DFSeriesExtended.priv.busy);
   50: XIC(Domino_internal_getMSG24.ER)XIC(DFSeriesExtended.GETMSG24.cmd.send)[CLR(DFSeriesExtended.GETMSG24.res.LEN) ,MOV(Domino_internal_getMSG24.EXERR,DFSeriesExtended.GETMSG24.error) ]OTU(DFSeriesExtended.GETMSG24.cmd.send)OTU(DFSeriesExtended.priv.busy)OTU(Domino_internal_getMSG24.ER);
   51: XIC(DFSeriesExtended.GETMSG25.cmd.send)XIO(Domino_internal_getMSG25.EN)XIO(DFSeriesExtended.priv.busy)OTE(DFSeriesExtended.priv.busy)MSG(Domino_internal_getMSG25);
   52: XIC(Domino_internal_getMSG25.DN)XIC(DFSeriesExtended.GETMSG25.cmd.send)CLR(DFSeriesExtended.GETMSG25.error)COP(DFSeriesExtended.priv.data[0],DFSeriesExtended.GETMSG25.res,1)OTU(DFSeriesExtended.GETMSG25.cmd.send)OTU(DFSeriesExtended.priv.busy);
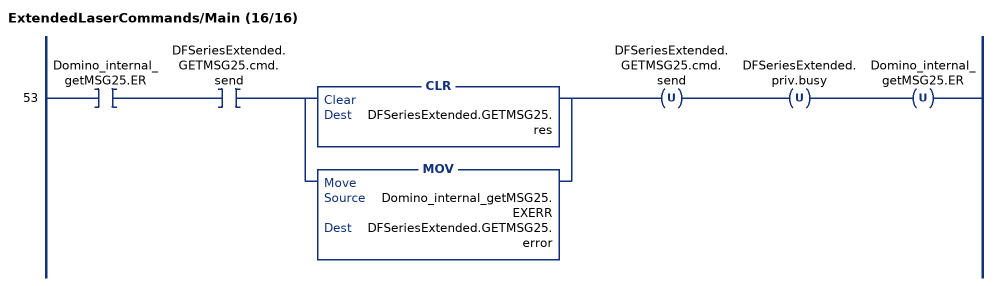
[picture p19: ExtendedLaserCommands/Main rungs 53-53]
   53: XIC(Domino_internal_getMSG25.ER)XIC(DFSeriesExtended.GETMSG25.cmd.send)[CLR(DFSeriesExtended.GETMSG25.res) ,MOV(Domino_internal_getMSG25.EXERR,DFSeriesExtended.GETMSG25.error) ]OTU(DFSeriesExtended.GETMSG25.cmd.send)OTU(DFSeriesExtended.priv.busy)OTU(Domino_internal_getMSG25.ER);
END_ROUTINE
END_PROGRAM
